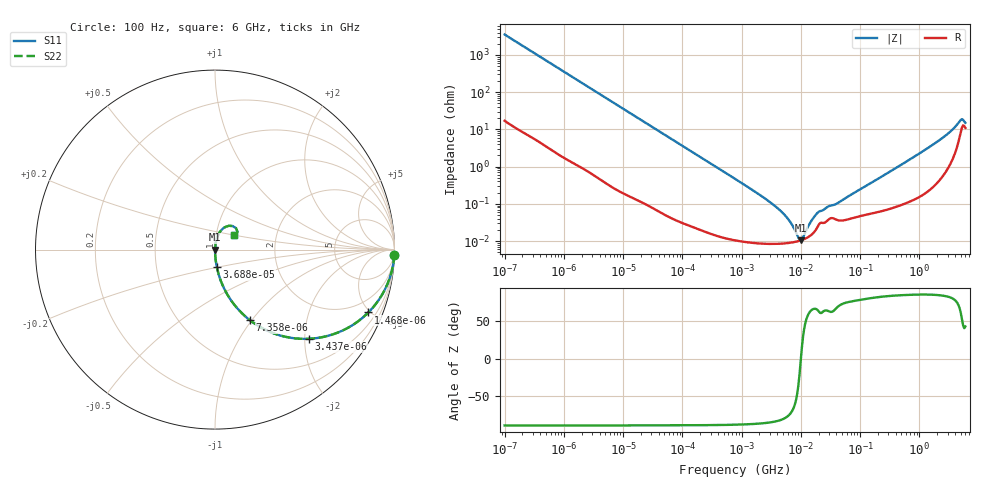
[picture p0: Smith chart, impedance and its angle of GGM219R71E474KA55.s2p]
!Murata Part Number: GGM219R71E474KA55
!These Parameters are Measured in Series Mode Connection
!Data Generated on Jun 19, 2026
!  o--ll--o
!Port1  Port2
!  o------o
!Operation Temp=25[degC], DC Bias Voltage=0[V]
!Freq. Start=100[Hz] Stop=6[GHz] 401[Steps]
# Hz S RI R 50
!Freq.(Hz) S11(Real) S11(Imag) S21(Real) S21(Imag) S12(Real) S12(Imag) S22(Real) S22(Imag)
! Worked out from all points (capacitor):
!   401 points, 100 Hz to 6 GHz, reference 50 ohm
!   read as one part in series: C = 448 nF near 109 Hz
!   lowest |Z| = 10.4 mohm at 9.942 MHz (marker M1)
!   series resonance near 10.03 MHz, so ESL is about 560 pH
!   S11 on the Smith chart (normalised r, x): 100 Hz: 1, -71; 1.468 kHz: 1.02, -4.88; 3.437 kHz: 1.01, -2.09; 7.358 kHz: 1.00, -0.98; 36.88 kHz: 1.00, -0.20; 6 GHz: 1.22, +0.21
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100  0.9991 -0.0281  0.000927 0.0281  0.000927 0.0281  0.9991 -0.0281
438  0.9845 -0.1209  0.0155 0.1209  0.0155 0.1209  0.9845 -0.1209
1468  0.8547 -0.3499  0.1453 0.3499  0.1453 0.3499  0.8547 -0.3499
2008  0.7597 -0.4247  0.2403 0.4247  0.2403 0.4247  0.7597 -0.4247
3437  0.5216 -0.4969  0.4784 0.4969  0.4784 0.4969  0.5216 -0.4969
7358  0.1942 -0.393  0.8058 0.393  0.8058 0.393  0.1942 -0.393
14402  0.0601 -0.2349  0.9399 0.2349  0.9399 0.2349  0.0601 -0.2349
36880  0.0102 -0.0971  0.9898 0.0971  0.9898 0.0971  0.0102 -0.0971
40335  0.00859 -0.0889  0.9914 0.0889  0.9914 0.0889  0.00859 -0.0889
774597  0.000127 -0.0047  0.9999 0.0047  0.9999 0.0047  0.000127 -0.0047
4440638  8.52e-05 -0.000667  0.9999 0.000667  0.9999 0.000667  8.52e-05 -0.000667
6353432  8.93e-05 -0.000348  0.9999 0.000348  0.9999 0.000348  8.93e-05 -0.000348
9090158  9.98e-05 -7.29e-05  0.9999 7.29e-05  0.9999 7.29e-05  9.98e-05 -7.29e-05
9941735  0.000104 -6.5e-06  0.9999 6.5e-06  0.9999 6.5e-06  0.000104 -6.5e-06
1.087309e7  0.00011 6e-05  0.9999 -6e-05  0.9999 -6e-05  0.00011 6e-05
1.555665e7  0.000154 0.000343  0.9998 -0.000343  0.9998 -0.000343  0.000154 0.000343
2.035112e7  0.000284 0.000554  0.9997 -0.000554  0.9997 -0.000554  0.000284 0.000554
4.165952e7  0.000367 0.000972  0.9996 -0.000972  0.9996 -0.000972  0.000367 0.000972
3.124326e8  0.000776 0.00714  0.9992 -0.00714  0.9992 -0.00714  0.000776 0.00714
2.142435e9  0.00655 0.0495  0.9934 -0.0495  0.9934 -0.0495  0.00655 0.0495
4.796499e9  0.078 0.1326  0.922 -0.1326  0.922 -0.1326  0.078 0.1326
6e9  0.1066 0.0833  0.8934 -0.0833  0.8934 -0.0833  0.1066 0.0833
